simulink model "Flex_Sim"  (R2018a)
settings: Solver=ode5  StartTime=0.0  StopTime=14000  FixedStep=Ts  MaxStep=0.000001  RelTol=1e-12  AbsTol=1e-8  EnableMultiTasking=on
InitFcn:
  | start
StopFcn:
  | pl
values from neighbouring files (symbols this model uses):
  Cw2b = [ 0,          0,          0    [start.m]    (also in run.m)
  d2r = pi/180    (= 0.0174532925199)    [start.m]    (also in run.m; runf.m; orbitic.m; Quan.m)
  Hmax = 10    [start.m]    (also in run.m)
  Jw = [Iw, 0, 0    [start.m]    (also in run.m)
  Kq1 = I22*ww^2 - 3*wo2*(I11-I33)    [start.m]    (also in run.m)
  Kq2 = 2*I22*zet*ww    [start.m]    (also in run.m)
  Kqi = 0.0005    [start.m]    (also in run.m)
  Kr1 = (0.1*I11*I33*zet^2/Hy0) - sqrt( ((0.01^zet^4*I11^2*I33^2)/Hy0^2)+(4*I11*I33*zet^2) )    [start.m]    (also in run.m)
  Kr2 = 0.05*Kr1    [start.m]    (also in run.m)
  Kr3 = 0.04*zet*(Kr2-Hy0) * sqrt(abs(Hy0/(I11*I33)))    [start.m]    (also in run.m)
  nt = 7    [start.m]    (also in run.m; runf.m)
  Tmax = 0.05    [start.m]    (also in run.m)
  Ts = 0.01    [start.m]    (also in run.m = 0.001; runf.m = 0.0005)
  wo = 0.00113    [start.m]    (also in run.m)
undefined symbols (not defined in the file or in its folder): Avf, Bvf, Cvf, den, DiscIntNeverNeededParam, dsen, Dvf, nsen, num, Phase_Plane, RW_Steering
libraries: simulink x5

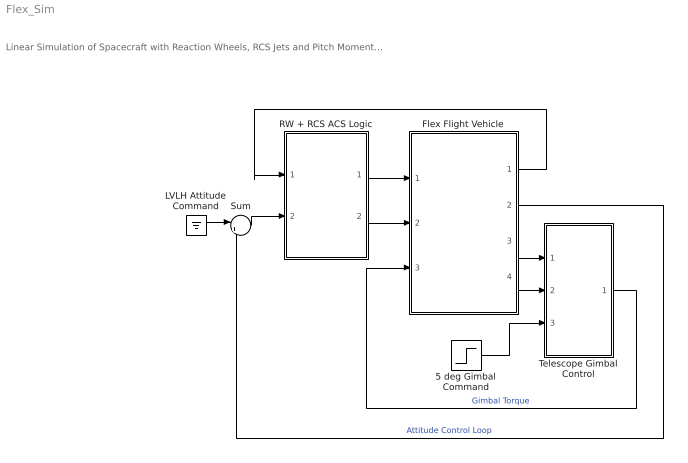
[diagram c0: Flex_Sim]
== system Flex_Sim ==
  note: Linear Simulation of Spacecraft with Reaction Wheels, RCS Jets and Pitch Momentum Bias
  5 deg Gimbal Command : Step  Time=20  After=[5, 5]*d2r  SampleTime=0
  Flex Flight Vehicle : Subsystem
  LVLH Attitude Command : Ground
  RW + RCS ACS Logic : Subsystem
  Sum : Sum  Inputs=|+-
  Telescope Gimbal Control : Subsystem
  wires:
  Flex Flight Vehicle/3(alfa) -> Telescope Gimbal Control/1(Gimb)
  Flex Flight Vehicle/4(alfad) -> Telescope Gimbal Control/2(Grate)
  Telescope Gimbal Control/1(GTrq) -> Flex Flight Vehicle/3(Tgimb)  "Gimbal Torque"
  RW + RCS ACS Logic/2(Trwi) -> Flex Flight Vehicle/2(Trw(i))
  Sum/1 -> RW + RCS ACS Logic/2(atter)
  Flex Flight Vehicle/2(atti) -> Sum/2  "Attitude Control Loop"
  RW + RCS ACS Logic/1(Frcs) -> Flex Flight Vehicle/1(Jet-7)
  Flex Flight Vehicle/1(Wr) -> RW + RCS ACS Logic/1(wr(i))
  5 deg Gimbal Command/1 -> Telescope Gimbal Control/3(Cmd)
  LVLH Attitude Command/1 -> Sum/1

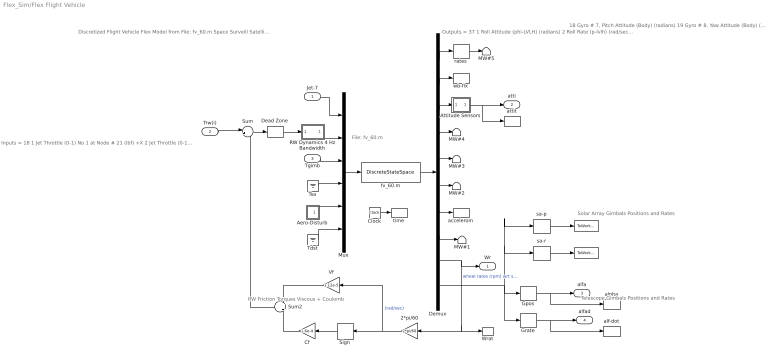
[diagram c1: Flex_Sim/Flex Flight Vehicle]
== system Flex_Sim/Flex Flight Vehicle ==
  note: Inputs = 18 1 Jet Throttle (0-1) No 1 at Node # 21 (lbf) +X 2 Jet Throttle (0-1) No 2 at Node # 22 (lbf) +X 3 Jet Throttle (0-1) No 3 at Node # 23 (lbf) +Y 4 Jet Throttle (0-1) No 4 at Node # 24 (lbf) -Y 5 Jet Throttle (0-1) No 5 at Node # 25 (lbf) -Y 6 Jet Throttle (0-1) No 6 at Node # 26 (lbf) +Y 7 Jet Throttle (0-1) No 7 at Node # 27 (lbf) +X 8 React-Wheel No 1 Torque to Spacecraft (ft-lb) 9 React-Wheel No 2 Torque to Spacecraft (ft-lb) 10 React-Wheel No 3 Torque to Spacecraft (ft-lb) 11 Elevation Trqu at Gimbal No 1 (ft-lb) 12 Azimuth Torque at Gimbal No 2 (ft-lb) 13 Rght SA Torque at Gimbal No 3 (ft-lb) 14 Left SA Torque at Gimbal No 4 (ft-lb) 15 Ext Torque Input 1 (ft-lb), dir: 1.00 0.00 0.00 16 Ext Torque Input 2 (ft-lb), dir: 0.00 1.00 0.00 17 Ext Torque Input 3 (ft-lb), dir: 0.00 0.00 1.00 18 Ext Torque Direct.=( 0.1970 -0.5964 -0.7782)
  note: Discretized Flight Vehicle Flex Model from File: fv_60.m Space Surveill Satellite with RCS and Reaction Wheels (Gimbals, 60 Modes, Z-Transf)
  note: Telescope Gimbals Positions and Rates
  note: Solar Array Gimbals Positions and Rates
  note: RW Friction Torques Viscous + Coulomb
  note: Outputs = 37 1 Roll Attitude (phi-LVLH) (radians) 2 Roll Rate (p-lvlh) (rad/sec) 3 Pitch Attitude (thet-LVLH) (radians) 4 Pitch Rate (q-lvlh) (rad/sec) 5 Yaw Attitude (psi-LVLH) (radians) 6 Yaw Rate (r-lvlh) (rad/sec) 7 Angle of attack, alfa, (radians) 8 Angle of sideslip, beta, (radian) 9 Change in Altitude, delta-h, (feet) 10 Forward Acceleration (V-dot) (ft/sec) 11 Cross Range Velocity (Vcr) (ft/sec) 12 Rate-Gyro # 1, Roll Rate (Body) (rad/sec) 13 Rate-Gyro # 2, Pitch Rate (Body) (rad/sec) 14 Rate-Gyro # 3, Yaw Rate (Body) (rad/sec) 15 Gyro # 4, Roll Attitude (Body) (radians) 16 Gyro # 5, Pitch Attitude (Body) (radians) 17 Gyro # 6, Yaw Attitude (Body) (radians)
  note: 18 Gyro # 7, Pitch Attitude (Body) (radians) 19 Gyro # 8, Yaw Attitude (Body) (radians) 20 Gyro # 9, Pitch Attitude (Body) (radians) 21 Gyro # 10, Yaw Attitude (Body) (radians) 22 Gyro # 11, Roll Attitude (Body) (radians) 23 Gyro # 12, Pitch Attitude (Body) (radians) 24 Gyro # 13, Yaw Attitude (Body) (radians) 25 Translat. Accelerom # 1, (along X), (ft/sec^2) 26 Translat. Accelerom # 2, (along Y), (ft/sec^2) 27 Reaction Wheel # 1 Rate (rpm) relative to vehicle 28 Reaction Wheel # 2 Rate (rpm) relative to vehicle 29 Reaction Wheel # 3 Rate (rpm) relative to vehicle 30 Rotation Angle at Elevati Gimbal No 1 31 Rotation Rate at Elevati Gimbal No 1 32 Rotation Angle at Azimuth Gimbal No 2 33 Rotation Rate at Azimuth Gimbal No 2 34 Rotation Angle at Rght SA Gimbal No 3 35 Rotation Rate at Rght SA Gimbal No 3 36 Rotation Angle at Left SA Gimbal No 4 37 Rotation Rate at Left SA Gimbal No 4
  note: File: fv_60.m
  Jet-7 : Inport
  Trw(i) : Inport  Port=2
  Tgimb : Inport  Port=3
  " " : ToWorkspace  VariableName=SA_pos  SampleTime=-1
  "   " : ToWorkspace  VariableName=SA_rate  SampleTime=-1
  2*pi/60 : Gain  Gain=2*pi/60
  Aero-Disturb : Subsystem
  Attitude Sensors : Subsystem
  Cf : Gain  Gain=1.6e-4
  Clock : Clock
  Dead Zone : DeadZone  LowerValue=-[1, 1]*Tmax/1000  UpperValue=[1 1]*Tmax/1000
  Demux : Demux  Outputs=[11, 3, 3, 2, 2, 3, 2, 1,2, 8]
  Gpos : Selector  InputPortWidth=8  IndexOptions=Index vector (dialog)  Indices=[1,3]  OutputSizes=1
  Grate : Selector  InputPortWidth=8  IndexOptions=Index vector (dialog)  Indices=[2, 4]  OutputSizes=1
  MW#{1..5} (5 alike) : Terminator
  Mux : Mux  Inputs=[7,3,2,2,3,1]
  RW Dynamics 4 Hz Bandwidth : Subsystem
  Sign : Signum
  Sum : Sum  Inputs=|+-
  Sum2 : Sum  Inputs=+|+
  Tdst : Ground
  Tsa : Ground
  Vf : Gain  Gain=1.12e-5
  Wrat : ToWorkspace  VariableName=wr  SampleTime=-1
  accelerom : ToWorkspace  VariableName=accel  SampleTime=-1
  alf-dot : ToWorkspace  VariableName=alfad  SampleTime=-1
  alpha : ToWorkspace  VariableName=alfa  SampleTime=-1
  attit : ToWorkspace  VariableName=atti  SampleTime=-1
  fv_60.m : DiscreteStateSpace  A=Avf  B=Bvf  C=Cvf  D=Dvf  SampleTime=Ts
  rates : Selector  InputPortWidth=11  IndexOptions=Index vector (dialog)  Indices=[2, 4, 6]  OutputSizes=1
  sa-p : Selector  InputPortWidth=8  IndexOptions=Index vector (dialog)  Indices=[5, 7]  OutputSizes=1
  sa-r : Selector  InputPortWidth=8  IndexOptions=Index vector (dialog)  Indices=[6, 8]  OutputSizes=1
  time : ToWorkspace  VariableName=time  SampleTime=-1
  wb-flx : ToWorkspace  VariableName=wb  SampleTime=-1
  Wr : Outport
  atti : Outport  Port=2
  alfa : Outport  Port=3
  alfad : Outport  Port=4
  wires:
  Mux/1 -> fv_60.m/1
  Demux/9 -> 2*pi/60/1, Wrat/1, Wr/1  "wheel rates (rpm) wrt spacecrft"
  Demux/1 -> rates/1
  Demux/10 -> Gpos/1, Grate/1, sa-p/1, sa-r/1
  Demux/2 -> wb-flx/1
  Demux/7 -> accelerom/1
  Demux/3 -> Attitude Sensors/1(I)
  Grate/1 -> alfad/1, alf-dot/1
  Gpos/1 -> alfa/1, alpha/1
  Tsa/1 -> Mux/4
  Tdst/1 -> Mux/6
  Clock/1 -> time/1
  Aero-Disturb/1(Td) -> Mux/5
  sa-p/1 -> " "/1
  sa-r/1 -> "   "/1
  Vf/1 -> Sum2/1
  Cf/1 -> Sum2/2
  Sign/1 -> Cf/1
  2*pi/60/1 -> Sign/1, Vf/1  "(rad/sec)"
  Tgimb/1 -> Mux/3
  fv_60.m/1 -> Demux/1
  Trw(i)/1 -> Sum/1
  Sum/1 -> Dead Zone/1
  Sum2/1 -> Sum/2
  Dead Zone/1 -> RW Dynamics 4 Hz Bandwidth/1(I)
  RW Dynamics 4 Hz Bandwidth/1(O) -> Mux/2
  Attitude Sensors/1(O) -> atti/1, attit/1
  Jet-7/1 -> Mux/1
  Demux/8 -> MW#1/1
  Demux/4 -> MW#4/1
  Demux/5 -> MW#3/1
  Demux/6 -> MW#2/1
  rates/1 -> MW#5/1

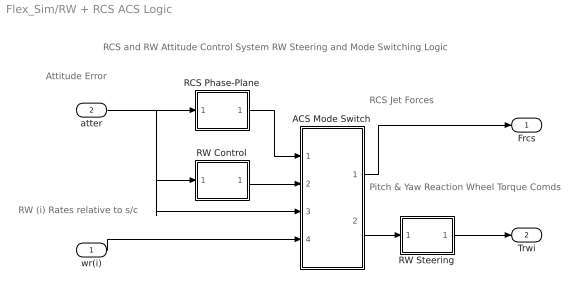
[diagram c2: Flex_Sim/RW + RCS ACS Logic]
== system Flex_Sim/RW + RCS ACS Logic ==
  note: RW (i) Rates relative to s/c
  note: Attitude Error
  note: Pitch & Yaw Reaction Wheel Torque Comds
  note: RCS Jet Forces
  note: RCS and RW Attitude Control System RW Steering and Mode Switching Logic
  wr(i) : Inport
  atter : Inport  Port=2
  ACS Mode Switch : Subsystem
  RCS Phase-Plane : Subsystem
  RW Control : Subsystem
  RW Steering : Subsystem
  Frcs : Outport
  Trwi : Outport  Port=2
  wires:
  atter/1 -> RCS Phase-Plane/1(atter), RW Control/1(atti), ACS Mode Switch/3(atter)
  ACS Mode Switch/2(" Trw") -> RW Steering/1(Trwc)
  wr(i)/1 -> ACS Mode Switch/4(wr(i))
  RCS Phase-Plane/1(f(nt)) -> ACS Mode Switch/1(Frcs)
  RW Steering/1(Twi) -> Trwi/1
  ACS Mode Switch/1(" Frcs") -> Frcs/1
  RW Control/1(Tc) -> ACS Mode Switch/2(Trw)

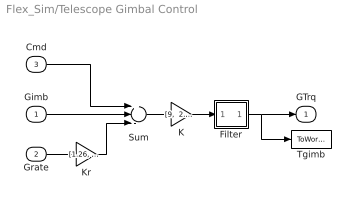
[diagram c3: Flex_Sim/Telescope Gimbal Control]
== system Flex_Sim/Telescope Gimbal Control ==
  Gimb : Inport
  Grate : Inport  Port=2
  Cmd : Inport  Port=3
  Filter : Subsystem
  K : Gain  Gain="[9,  2.85]"
  Kr : Gain  Gain="[1.26,  1.14]"
  Sum : Sum  Inputs=+--
  Tgimb : ToWorkspace  VariableName=Tgimb  SampleTime=-1
  GTrq : Outport
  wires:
  Sum/1 -> K/1
  Gimb/1 -> Sum/2
  Grate/1 -> Kr/1
  K/1 -> Filter/1(I)
  Kr/1 -> Sum/3
  Cmd/1 -> Sum/1
  Filter/1(O) -> GTrq/1, Tgimb/1

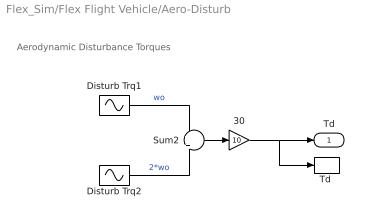
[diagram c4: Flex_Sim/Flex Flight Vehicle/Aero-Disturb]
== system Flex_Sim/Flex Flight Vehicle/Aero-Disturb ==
  note: Aerodynamic Disturbance Torques
  30 : Gain  Gain=10
  Disturb Trq1 : Sin  Amplitude="[0.0,   1,   0.2]*0.0001"  Bias="[0.0,  0.5,  0.15]*0.0001"  Frequency=[wo, wo, wo]  SampleTime=0
  Disturb Trq2 : Sin  Amplitude=[0, 1.2, 1]*0.0001  Bias="[0  0.1 0.1]*0.0001"  Frequency=[wo, wo, wo]*2  SampleTime=0
  Sum2 : Sum  Inputs=+|+
  "Td " : ToWorkspace  VariableName=Td  SampleTime=-1
  Td : Outport
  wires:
  30/1 -> "Td "/1, Td/1
  Disturb Trq2/1 -> Sum2/2  "2*wo"
  Sum2/1 -> 30/1
  Disturb Trq1/1 -> Sum2/1  "wo"

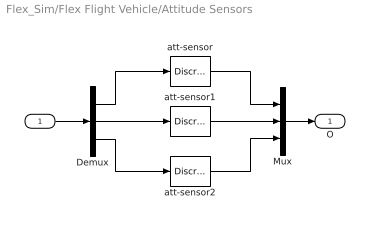
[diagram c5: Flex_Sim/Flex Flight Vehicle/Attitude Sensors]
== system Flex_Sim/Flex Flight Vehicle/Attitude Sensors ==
  I : Inport
  Demux : Demux  Outputs=3
  Mux : Mux  Inputs=3
  att-sensor : DiscreteTransferFcn  Numerator=[nsen]  Denominator=[dsen]  SampleTime=Ts
  att-sensor1 : DiscreteTransferFcn  Numerator=[nsen]  Denominator=[dsen]  SampleTime=Ts
  att-sensor2 : DiscreteTransferFcn  Numerator=[nsen]  Denominator=[dsen]  SampleTime=Ts
  O : Outport
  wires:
  I/1 -> Demux/1
  Mux/1 -> O/1
  att-sensor/1 -> Mux/1
  Demux/1 -> att-sensor/1
  Demux/3 -> att-sensor2/1
  att-sensor2/1 -> Mux/3
  Demux/2 -> att-sensor1/1
  att-sensor1/1 -> Mux/2

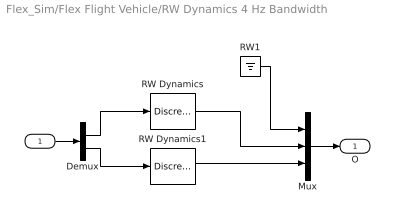
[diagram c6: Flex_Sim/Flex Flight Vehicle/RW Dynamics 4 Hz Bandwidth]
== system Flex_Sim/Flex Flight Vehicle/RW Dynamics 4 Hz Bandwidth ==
  I : Inport
  Demux : Demux  Outputs=2
  Mux : Mux  Inputs=3
  RW Dynamics : DiscreteTransferFcn  Numerator="[0  0.221199217]"  Denominator=[1 -0.778800783]  SampleTime=Ts
  RW Dynamics1 : DiscreteTransferFcn  Numerator="[0  0.221199217]"  Denominator=[1 -0.778800783]  SampleTime=Ts
  RW1 : Ground
  O : Outport
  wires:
  Demux/2 -> RW Dynamics1/1
  Demux/1 -> RW Dynamics/1
  RW Dynamics/1 -> Mux/2
  RW Dynamics1/1 -> Mux/3
  I/1 -> Demux/1
  Mux/1 -> O/1
  RW1/1 -> Mux/1

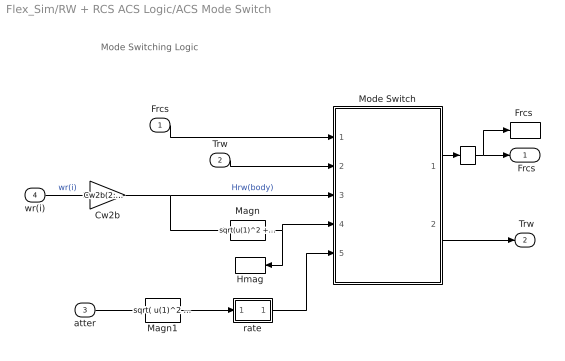
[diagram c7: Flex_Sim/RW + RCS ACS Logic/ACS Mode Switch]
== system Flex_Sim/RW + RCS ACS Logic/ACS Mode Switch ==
  note: Mode Switching Logic
  Frcs : Inport
  Trw : Inport  Port=2
  atter : Inport  Port=3
  wr(i) : Inport  Port=4
  "   " : Memory
  Cw2b : Gain  Gain=Cw2b(2:3,2:3)*Jw(2:3,2:3)  Multiplication=Matrix(K*u)
  "Frcs " : ToWorkspace  VariableName=Frcs  SampleTime=-1
  Hmag : ToWorkspace  VariableName=Hmag  SampleTime=-1
  Magn : Fcn  Expr=sqrt(u(1)^2 + u(2)^2)
  Magn1 : Fcn  Expr=sqrt( u(1)^2 + u(2)^2 + u(3)^2 )
  Mode Switch : Stateflow chart  TreatAsAtomicUnit=on
  rate : Subsystem
  " Frcs" : Outport
  " Trw" : Outport  Port=2
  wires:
  wr(i)/1 -> Cw2b/1  "wr(i)"
  Frcs/1 -> Mode Switch/1(Fi)
  Trw/1 -> Mode Switch/2(Tci)
  atter/1 -> Magn1/1
  Magn/1 -> Mode Switch/4(hmag), Hmag/1
  Mode Switch/1(Fo) -> "   "/1
  Mode Switch/2(Tco) -> " Trw"/1
  Cw2b/1 -> Mode Switch/3(hrwa), Magn/1  "Hrw(body)"
  Magn1/1 -> rate/1(in)
  rate/1(ou) -> Mode Switch/5(atter)
  "   "/1 -> "Frcs "/1, " Frcs"/1

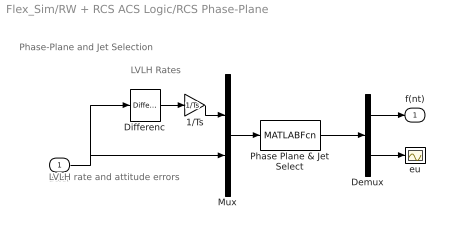
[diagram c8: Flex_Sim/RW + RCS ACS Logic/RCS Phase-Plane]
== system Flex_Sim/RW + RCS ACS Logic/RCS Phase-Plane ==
  note: LVLH Rates
  note: LVLH rate and attitude errors
  note: Phase-Plane and Jet Selection
  atter : Inport
  1/Ts : Gain  Gain=1/Ts
  Demux : Demux  Outputs=[nt, 3]
  Differenc : simulink/Discrete/Difference  ICPrevInput=0.0  InputProcessing=Inherited  OutMin=[]  OutMax=[]  OutDataType=sfix(16)  OutScaling=2^-10  DoSatur=off
  Mux : Mux  Inputs="[3  3]"
  Phase Plane & Jet Select : MATLABFcn  MATLABFcn=Phase_Plane( u(1:3), u(4:6) )  OutputDimensions=nt + 3
  eu : Scope
  f(nt) : Outport
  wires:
  Differenc/1 -> 1/Ts/1
  Mux/1 -> Phase Plane & Jet Select/1
  Phase Plane & Jet Select/1 -> Demux/1
  Demux/1 -> f(nt)/1
  Demux/2 -> eu/1
  1/Ts/1 -> Mux/1
  atter/1 -> Differenc/1, Mux/2

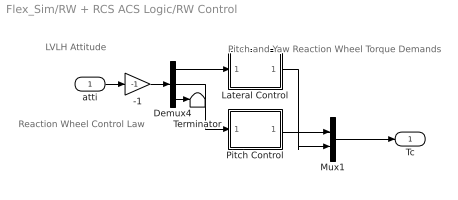
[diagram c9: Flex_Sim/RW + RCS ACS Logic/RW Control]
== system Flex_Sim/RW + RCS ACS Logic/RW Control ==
  note: Reaction Wheel Control Law
  note: LVLH Attitude
  note: Pitch and Yaw Reaction Wheel Torque Demands
  atti : Inport
  -1 : Gain  Gain=-1
  Demux4 : Demux  Outputs=3
  Lateral Control : Subsystem
  Mux1 : Mux  Inputs=2
  Pitch Control : Subsystem
  Terminator : Terminator
  Tc : Outport
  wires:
  Mux1/1 -> Tc/1
  Lateral Control/1(Tcz) -> Mux1/2
  -1/1 -> Demux4/1
  atti/1 -> -1/1
  Demux4/2 -> Pitch Control/1(the)
  Pitch Control/1(Tcy) -> Mux1/1
  Demux4/1 -> Lateral Control/1(phi)
  Demux4/3 -> Terminator/1

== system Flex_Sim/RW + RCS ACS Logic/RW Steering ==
  note: RW (i) Torque Commands
  note: Reaction Wheel Steering Logic
  Trwc : Inport
  Demux : Demux  Outputs=[2, 1]
  RW Steering : MATLABFcn  MATLABFcn=RW_Steering( u(1:2) )  OutputDimensions=3
  Trw : ToWorkspace  VariableName=Trw  SampleTime=-1
  Twm : Scope
  Twi : Outport
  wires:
  Demux/2 -> Twm/1
  Demux/1 -> Trw/1, Twi/1
  RW Steering/1 -> Demux/1
  Trwc/1 -> RW Steering/1  "RW torque cmd (pitch & yaw)"

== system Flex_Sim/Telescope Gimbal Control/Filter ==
  I : Inport
  Demux : Demux  Outputs=2
  Filter1 : TransferFcn  Numerator=[80]  Denominator=[1 80]
  Filter2 : TransferFcn  Numerator=[80]  Denominator=[1 80]
  Mux : Mux  Inputs=2
  O : Outport
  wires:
  Mux/1 -> O/1
  I/1 -> Demux/1
  Demux/2 -> Filter2/1
  Demux/1 -> Filter1/1
  Filter2/1 -> Mux/2
  Filter1/1 -> Mux/1

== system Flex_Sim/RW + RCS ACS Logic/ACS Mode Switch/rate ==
  in : Inport
  1/Ts : Gain  Gain=1/Ts
  Abs : Abs
  Differenc : simulink/Discrete/Difference  ICPrevInput=0.0  InputProcessing=Inherited  OutMin=[]  OutMax=[]  OutDataType=sfix(16)  OutScaling=2^-10  DoSatur=off
  ou : Outport
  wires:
  Differenc/1 -> 1/Ts/1
  1/Ts/1 -> Abs/1
  in/1 -> Differenc/1
  Abs/1 -> ou/1

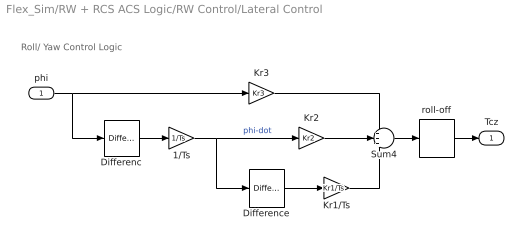
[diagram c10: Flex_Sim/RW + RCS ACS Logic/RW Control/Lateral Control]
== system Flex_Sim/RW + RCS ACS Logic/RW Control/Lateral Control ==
  note: Roll/ Yaw Control Logic
  phi : Inport
  1/Ts : Gain  Gain=1/Ts
  Differenc : simulink/Discrete/Difference  ICPrevInput=0.0  InputProcessing=Inherited  OutMin=[]  OutMax=[]  OutDataType=sfix(16)  OutScaling=2^-10  DoSatur=off
  Difference : simulink/Discrete/Difference  ICPrevInput=0.0  InputProcessing=Inherited  OutMin=[]  OutMax=[]  OutDataType=sfix(16)  OutScaling=2^-10  DoSatur=off
  Kr1/Ts : Gain  Gain=Kr1/Ts
  Kr2 : Gain  Gain=Kr2
  Kr3 : Gain  Gain=Kr3
  Sum4 : Sum  Inputs=+++
  roll-off : DiscreteTransferFcn  Numerator=[num]  Denominator=[den]  SampleTime=Ts
  Tcz : Outport
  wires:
  roll-off/1 -> Tcz/1
  1/Ts/1 -> Difference/1, Kr2/1  "phi-dot"
  Differenc/1 -> 1/Ts/1
  Difference/1 -> Kr1/Ts/1
  Sum4/1 -> roll-off/1
  phi/1 -> Differenc/1, Kr3/1
  Kr1/Ts/1 -> Sum4/3
  Kr2/1 -> Sum4/2
  Kr3/1 -> Sum4/1

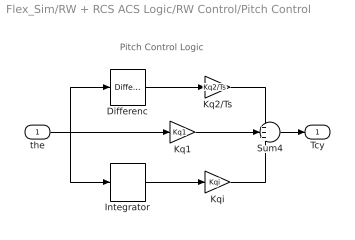
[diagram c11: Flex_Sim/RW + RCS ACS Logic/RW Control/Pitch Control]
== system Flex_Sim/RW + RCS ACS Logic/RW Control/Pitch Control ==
  note: Pitch Control Logic
  the : Inport
  Differenc : simulink/Discrete/Difference  ICPrevInput=0.0  InputProcessing=Inherited  OutMin=[]  OutMax=[]  OutDataType=sfix(16)  OutScaling=2^-10  DoSatur=off
  Integrator : DiscreteIntegrator  SampleTime=Ts  ICPrevOutput=DiscIntNeverNeededParam  ICPrevScaledInput=DiscIntNeverNeededParam
  Kq1 : Gain  Gain=Kq1
  Kq2/Ts : Gain  Gain=Kq2/Ts
  Kqi : Gain  Gain=Kqi
  Sum4 : Sum  Inputs=+++
  Tcy : Outport
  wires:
  Differenc/1 -> Kq2/Ts/1
  Integrator/1 -> Kqi/1
  Kqi/1 -> Sum4/3
  the/1 -> Differenc/1, Integrator/1, Kq1/1
  Kq2/Ts/1 -> Sum4/1
  Sum4/1 -> Tcy/1
  Kq1/1 -> Sum4/2

== stateflow chart Flex_Sim/RW + RCS
ACS Logic/ACS Mode 
Switch/Mode Switch ==
  state RCS1
    en:Fo=Fi;
    en:Tco=-hrwa*Tmax/hmag;
  state RCS2
    en:Fo=Fi;
    en:Tco=Tz;
  state RW
    en:Fo=Fz;
    en:Tco=Tci;
  RCS2 -> RCS1 : [hmag>Hmax/10]
  RCS1 -> RCS1 : [hmag>=Hmax/10 ... || atter>=Rlim]
  RCS1 -> (junction 13)
  (junction 13) -> RCS2
  (junction 13) -> RW : [hmag<Hmax/10 ... && atter<Rlim]
  RW -> RCS1 : [hmag>=Hmax]
  RCS2 -> RW : [atter<Rlim]
  (default) -> RW
  RW -> RW : [hmag<Hmax]
  data: Fi input; Tci input; Fo output double; Tco output double; Tmax parameter double; Hmax parameter double; hrwa input; hmag input; Fz constant double; atter input; Tz constant double; Rlim constant double =0.8e-3
